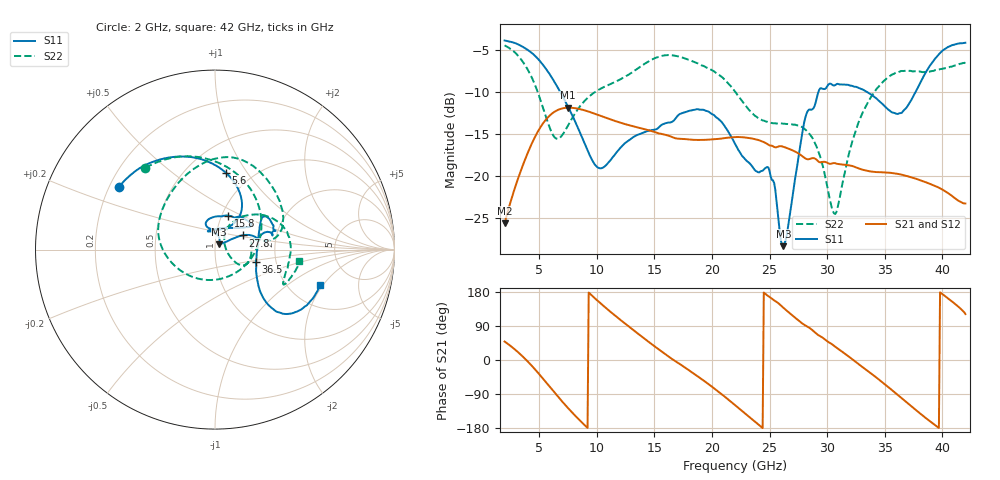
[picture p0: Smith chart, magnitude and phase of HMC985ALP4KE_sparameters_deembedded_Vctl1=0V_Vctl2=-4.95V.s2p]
!s2p File: Measurements: S11, S21, S12, S22
# GHz S dB R 50.0
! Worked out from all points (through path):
!   401 points, 2 GHz to 42 GHz, reference 50 ohm
!   highest |S21| = -11.90 dB at 7.5 GHz (marker M1); lowest = -25.7 dB at 2 GHz (marker M2)
!   lowest |S11| = -28.4 dB at 26.2 GHz (marker M3), VSWR 1.08, Z = 52.2 + j3.17 ohm
!   |S11| at or under -10 dB: 6.819 GHz to 29.25 GHz (22.43 GHz wide, 124 % of centre); 33.42 GHz to 37.69 GHz (4.266 GHz wide, 12 % of centre)
!   |S22| runs from -24.6 to -4.5 dB; largest |S21 - S12| = 0.00024
!   S11 on the Smith chart (normalised r, x): 2 GHz: 0.24, +0.28; 5.6 GHz: 0.76, +0.80; 15.8 GHz: 1.07, +0.42; 27.8 GHz: 1.34, +0.22; 36.5 GHz: 1.57, -0.23; 42 GHz: 2.93, -1.89
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2  -3.88 147.0  -25.66 48.7  -25.67 48.6  -4.47 130.5
3.6  -4.66 120.3  -18.70 8.4  -18.70 8.4  -6.47 84.9
4.7  -5.80 99.5  -15.22 -26.8  -15.22 -26.8  -9.40 43.4
5.6  -7.29 81.9  -13.30 -59.0  -13.30 -59.0  -13.02 -3.6
6.5  -9.22 66.5  -12.25 -91.9  -12.25 -91.9  -15.59 -68.6
7.5  -11.76 55.4  -11.90 -126.7  -11.90 -126.7  -14.03 -131.1
8.7  -15.38 55.1  -12.12 -164.6  -12.12 -164.6  -11.46 -170.1
10.4  -19.12 89.6  -12.90 147.6  -12.90 147.6  -9.59 162.6
15.4  -14.23 75.6  -14.97 27.7  -14.97 27.7  -5.82 87.4
15.8  -13.84 68.7  -15.07 18.8  -15.08 18.8  -5.68 82.3
19.4  -12.23 33.3  -15.73 -57.0  -15.73 -57.0  -7.02 35.4
22  -16.18 51.0  -15.40 -119.0  -15.41 -119.0  -9.97 9.8
24.9  -19.03 104.8  -16.32 168.3  -16.33 168.3  -13.62 13.2
26.2  -28.41 52.9  -16.56 137.9  -16.56 137.9  -13.81 -2.1
27.8  -15.23 27.2  -17.63 97.4  -17.63 97.4  -14.20 -24.0
28.7  -12.11 12.5  -17.92 79.3  -17.93 79.2  -15.46 -31.0
30.7  -9.21 20.7  -18.51 35.0  -18.52 35.0  -24.57 19.7
32.8  -9.58 33.9  -19.17 -12.6  -19.17 -12.6  -13.38 53.7
35.4  -12.21 11.8  -19.65 -73.8  -19.65 -73.8  -8.18 21.9
36.5  -12.48 -16.7  -19.89 -101.6  -19.91 -101.6  -7.52 7.8
39.5  -5.85 -43.9  -21.31 -174.9  -21.32 -174.9  -7.40 -26.4
42  -4.16 -18.7  -23.32 121.2  -23.32 121.2  -6.50 -7.5
